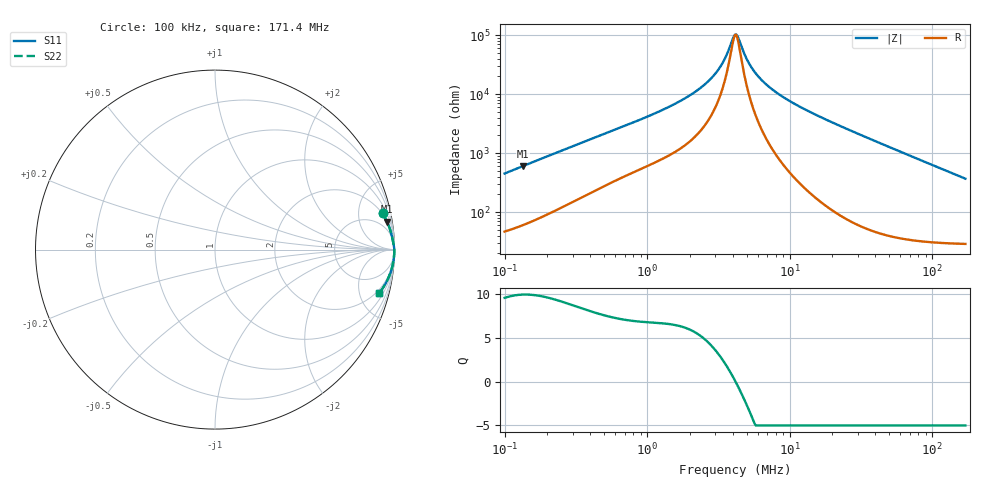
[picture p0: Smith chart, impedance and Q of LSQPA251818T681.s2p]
! LSQPA251818T681  S-PARAMETER MODEL  ( General Type )
! Model Generated by TAIYO YUDEN Corporation (http://www.ty-top.com)
! Version 3.0
! TAIYO YUDEN Control No. 160907NF25SB-FAC
! Copyright(c) 2007 TAIYO YUDEN CO.,LTD. All Rights Reserved.
! Product Description (link to TY-COMPAS)
! https://ds.yuden.co.jp/TYCOMPAS/or/detail?pn=LSQPA251818T681K&u=M
! Products Name : Inductors
! Characteristics :
!  Inductance : 680 uH , SRF(min) : 3.0 MHz , DC Resistance(max) : 36.4 Ohm
!  Rated Current : Saturation :65 mA , Temp Rise : 60 mA (40 degC)
!  Case Size : 2.5 x 1.8 / 0.098 x 0.071 [mm/inch] , Thickness : 1.8 / 0.071 [mm/inch]
!  (Conditions: Temperature = 25 degC , DC Bias Current/Voltage = 0A / 0V)
! External Node Assignments :
!  1  o---GGG---o  2
! GND o---------o GND
! Frequency Range : 0.1MHz  -  171.398534MHz  [ 402 STEP ]
# MHz S RI R 50
! Freq[MHz].  S11 Real  S11 Imag  S21 Real  S21 Imag  S12 Real  S12 Imag  S22 Real  S22 Imag
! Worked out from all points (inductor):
!   401 points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, 100 kHz to 171.4 MHz, reference 50 ohm
!   read as one part in series: L = 710 uH near 103.8 kHz
!   highest Q = 9.95 at 134.7 kHz (marker M1), where L = 710 uH
!   self-resonance near 4.14 MHz
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0.1  0.9342 0.2012  0.0658 -0.2012  0.0658 -0.2012  0.9342 0.2012
0.134698  0.9585 0.1554  0.0415 -0.1554  0.0415 -0.1554  0.9585 0.1554
0.348094  0.9879 0.0649  0.0121 -0.0649  0.0121 -0.0649  0.9879 0.0649
1.211692  0.9967 0.0194  0.00329 -0.0194  0.00329 -0.0194  0.9967 0.0194
1.966087  0.9981 0.0106  0.00188 -0.0106  0.00188 -0.0106  0.9981 0.0106
2.368389  0.9985 0.00772  0.00154 -0.00772  0.00154 -0.00772  0.9985 0.00772
2.748737  0.9987 0.00559  0.00133 -0.00559  0.00133 -0.00559  0.9987 0.00559
3.073571  0.9988 0.00406  0.0012 -0.00406  0.0012 -0.00406  0.9988 0.00406
3.373404  0.9989 0.00281  0.00112 -0.00281  0.00112 -0.00281  0.9989 0.00281
3.634197  0.9989 0.00183  0.00106 -0.00183  0.00106 -0.00183  0.9989 0.00183
3.98872  0.999 0.000607  0.001 -0.000607  0.001 -0.000607  0.999 0.000607
4.140031  0.999 0.000119  0.00098 -0.000119  0.00098 -0.000119  0.999 0.000119
4.217825  0.999 -0.000126  0.00097 0.000126  0.00097 0.000126  0.999 -0.000126
4.377827  0.999 -0.000615  0.000953 0.000615  0.000953 0.000615  0.999 -0.000615
4.895181  0.9991 -0.00209  0.000911 0.00209  0.000911 0.00209  0.9991 -0.00209
5.372715  0.9991 -0.00335  0.000888 0.00335  0.000888 0.00335  0.9991 -0.00335
6.472082  0.9991 -0.00596  0.000869 0.00596  0.000869 0.00596  0.9991 -0.00596
8.881561  0.9991 -0.0109  0.000925 0.0109  0.000925 0.0109  0.9991 -0.0109
14.41119  0.9987 -0.0209  0.00129 0.0209  0.00129 0.0209  0.9987 -0.0209
50.16444  0.9914 -0.0781  0.00862 0.0781  0.00862 0.0781  0.9914 -0.0781
101.7716  0.9674 -0.1544  0.0326 0.1544  0.0326 0.1544  0.9674 -0.1544
171.3985  0.9151 -0.2422  0.0849 0.2422  0.0849 0.2422  0.9151 -0.2422
